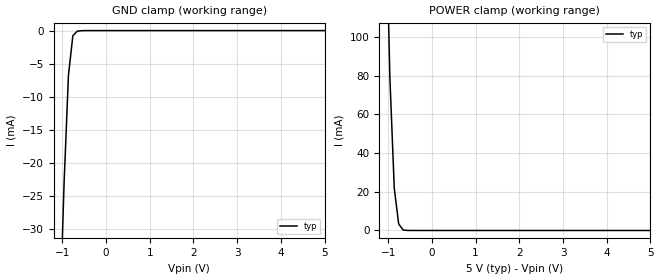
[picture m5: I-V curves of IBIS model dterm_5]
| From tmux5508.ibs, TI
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| dterm_5
[Model]   dterm_5
Model_type   Terminator
|   typ   min   max
C_comp   1.008417e-11   NA   NA
[Voltage Range]   5   NA   NA
[Temperature Range]   27   NA   NA
[Power Clamp Reference]   5   NA   NA
[GND Clamp Reference]   0   NA   NA
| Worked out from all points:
|   GND clamp passes 1 mA (typ) near -0.76 V on its own axis
|   POWER clamp passes 1 mA (typ) near -0.68 V on its own axis
[GND Clamp]
|   Voltage   I(typ)   I(min)   I(max)
-5V       -2.839A    NA         NA
-1.061V   -45mA      NA         NA
-959.6mV  -23.25mA   NA         NA
-858.6mV  -6.731mA   NA         NA
-757.6mV  -768.2uA   NA         NA
-656.6mV  -81.6uA    NA         NA
5V        469.4pA    NA         NA
[POWER Clamp]
|   Voltage   I(typ)   I(min)   I(max)
-5V       8.447A     NA         NA
-1.061V   178.6mA    NA         NA
-959.6mV  79.51mA    NA         NA
-858.6mV  21.79mA    NA         NA
-757.6mV  3.38mA     NA         NA
-656.6mV  255.5uA    NA         NA
5V        -576.6pA   NA         NA
